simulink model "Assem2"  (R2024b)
settings: Solver=VariableStepAuto  StartTime=0.0  StopTime=10.0  RelTol=1e-3
undefined symbols (not defined in the file or in its folder): deg, kg, m, mm, N, s, smiData, X, Y, Z
libraries: sm_lib x14

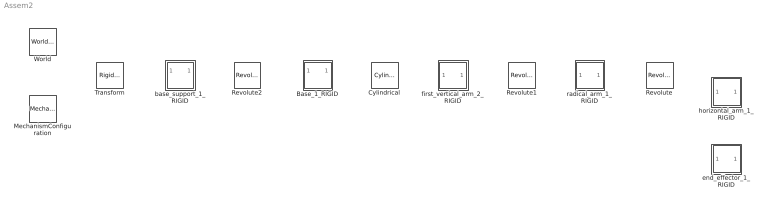
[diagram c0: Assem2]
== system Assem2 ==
  Base_1_RIGID : Subsystem
  Cylindrical : sm_lib/Joints/Cylindrical Joint  JointMode=Normal  CompositeWrenchDir=FollowerOnBase  CompositeWrenchFrame=BaseFrame  SenseConstraintForce=off  SenseConstraintTorque=off  SenseTotalForce=off  SenseTotalTorque=off  RzPositionTargetSpecify=on  RzPositionTargetPriority=Low  RzPositionTargetValue=smiData.CylindricalJoint(1).Rz.Pos  RzPositionTargetValueUnits=deg  RzVelocityTargetSpecify=off  RzVelocityTargetPriority=High  RzVelocityTargetValue=0  RzVelocityTargetValueUnits=deg/s  RzEquilibriumPosition=0  RzEquilibriumPositionUnits=deg  RzSpringStiffness=0  RzSpringStiffnessUnits=N*m/deg  RzDampingCoefficient=0  RzDampingCoefficientUnits=N*m/(deg/s)  RzLowerLimitSpecify=off  RzLowerLimitBound=-90  RzLowerLimitBoundUnits=deg  RzLowerLimitStiffness=1e4  RzLowerLimitStiffnessUnits=N*m/deg  RzLowerLimitDamping=10  RzLowerLimitDampingUnits=N*m/(deg/s)  RzLowerLimitTransitionRegionWidth=0.1  RzLowerLimitTransitionRegionWidthUnits=deg  RzUpperLimitSpecify=off  RzUpperLimitBound=90  RzUpperLimitBoundUnits=deg  RzUpperLimitStiffness=1e4  RzUpperLimitStiffnessUnits=N*m/deg  RzUpperLimitDamping=10  RzUpperLimitDampingUnits=N*m/(deg/s)  RzUpperLimitTransitionRegionWidth=0.1  RzUpperLimitTransitionRegionWidthUnits=deg  RzTorqueActuationMode=NoTorque  RzMotionActuationMode=ComputedMotion  RzSensePosition=off  RzSenseVelocity=off  RzSenseAcceleration=off  RzSenseTorqueForce=off  RzSenseLowerLimitTorqueForce=off  RzSenseUpperLimitTorqueForce=off  PzPositionTargetSpecify=on  PzPositionTargetPriority=Low  PzPositionTargetValue=smiData.CylindricalJoint(1).Pz.Pos  PzPositionTargetValueUnits=mm  PzVelocityTargetSpecify=off  PzVelocityTargetPriority=High  PzVelocityTargetValue=0  PzVelocityTargetValueUnits=m/s  PzEquilibriumPosition=0  PzEquilibriumPositionUnits=m  PzSpringStiffness=0  PzSpringStiffnessUnits=N/m  PzDampingCoefficient=0  PzDampingCoefficientUnits=N/(m/s)  PzLowerLimitSpecify=off  PzLowerLimitBound=-1  PzLowerLimitBoundUnits=m  PzLowerLimitStiffness=1e6  PzLowerLimitStiffnessUnits=N/m  PzLowerLimitDamping=1e3  PzLowerLimitDampingUnits=N/(m/s)  PzLowerLimitTransitionRegionWidth=1e-4  PzLowerLimitTransitionRegionWidthUnits=m  PzUpperLimitSpecify=off  PzUpperLimitBound=1  PzUpperLimitBoundUnits=m  PzUpperLimitStiffness=1e6  PzUpperLimitStiffnessUnits=N/m  PzUpperLimitDamping=1e3  PzUpperLimitDampingUnits=N/(m/s)  PzUpperLimitTransitionRegionWidth=1e-4  PzUpperLimitTransitionRegionWidthUnits=m  PzTorqueActuationMode=NoTorque  PzMotionActuationMode=ComputedMotion  PzSensePosition=off  PzSenseVelocity=off  PzSenseAcceleration=off  PzSenseTorqueForce=off  PzSenseLowerLimitTorqueForce=off  PzSenseUpperLimitTorqueForce=off
  MechanismConfiguration : sm_lib/Utilities/Mechanism Configuration  UniformGravity=Constant  GravityVector=[0 -9.80665 0]  GravityVectorUnits=m/s^2  LinearizationDelta=0.001  JointModeTransitionNonlinearIterations=2
  Revolute : sm_lib/Joints/Revolute Joint  JointMode=Normal  CompositeWrenchDir=FollowerOnBase  CompositeWrenchFrame=BaseFrame  SenseConstraintForce=off  SenseConstraintTorque=off  SenseTotalForce=off  SenseTotalTorque=off  PositionTargetSpecify=on  PositionTargetPriority=Low  PositionTargetValue=smiData.RevoluteJoint(1).Rz.Pos  PositionTargetValueUnits=deg  VelocityTargetSpecify=off  VelocityTargetPriority=High  VelocityTargetValue=0  VelocityTargetValueUnits=deg/s  EquilibriumPosition=0  EquilibriumPositionUnits=deg  SpringStiffness=0  SpringStiffnessUnits=N*m/deg  DampingCoefficient=0  DampingCoefficientUnits=N*m/(deg/s)  LowerLimitSpecify=off  LowerLimitBound=-90  LowerLimitBoundUnits=deg  LowerLimitStiffness=1e4  LowerLimitStiffnessUnits=N*m/deg  LowerLimitDamping=10  LowerLimitDampingUnits=N*m/(deg/s)  LowerLimitTransitionRegionWidth=0.1  LowerLimitTransitionRegionWidthUnits=deg  UpperLimitSpecify=off  UpperLimitBound=90  UpperLimitBoundUnits=deg  UpperLimitStiffness=1e4  UpperLimitStiffnessUnits=N*m/deg  UpperLimitDamping=10  UpperLimitDampingUnits=N*m/(deg/s)  UpperLimitTransitionRegionWidth=0.1  UpperLimitTransitionRegionWidthUnits=deg  TorqueActuationMode=NoTorque  MotionActuationMode=ComputedMotion  SensePosition=off  SenseVelocity=off  SenseAcceleration=off  SenseTorqueForce=off  SenseLowerLimitTorqueForce=off  SenseUpperLimitTorqueForce=off
  Revolute1 : sm_lib/Joints/Revolute Joint  JointMode=Normal  CompositeWrenchDir=FollowerOnBase  CompositeWrenchFrame=BaseFrame  SenseConstraintForce=off  SenseConstraintTorque=off  SenseTotalForce=off  SenseTotalTorque=off  PositionTargetSpecify=on  PositionTargetPriority=Low  PositionTargetValue=smiData.RevoluteJoint(2).Rz.Pos  PositionTargetValueUnits=deg  VelocityTargetSpecify=off  VelocityTargetPriority=High  VelocityTargetValue=0  VelocityTargetValueUnits=deg/s  EquilibriumPosition=0  EquilibriumPositionUnits=deg  SpringStiffness=0  SpringStiffnessUnits=N*m/deg  DampingCoefficient=0  DampingCoefficientUnits=N*m/(deg/s)  LowerLimitSpecify=off  LowerLimitBound=-90  LowerLimitBoundUnits=deg  LowerLimitStiffness=1e4  LowerLimitStiffnessUnits=N*m/deg  LowerLimitDamping=10  LowerLimitDampingUnits=N*m/(deg/s)  LowerLimitTransitionRegionWidth=0.1  LowerLimitTransitionRegionWidthUnits=deg  UpperLimitSpecify=off  UpperLimitBound=90  UpperLimitBoundUnits=deg  UpperLimitStiffness=1e4  UpperLimitStiffnessUnits=N*m/deg  UpperLimitDamping=10  UpperLimitDampingUnits=N*m/(deg/s)  UpperLimitTransitionRegionWidth=0.1  UpperLimitTransitionRegionWidthUnits=deg  TorqueActuationMode=NoTorque  MotionActuationMode=ComputedMotion  SensePosition=off  SenseVelocity=off  SenseAcceleration=off  SenseTorqueForce=off  SenseLowerLimitTorqueForce=off  SenseUpperLimitTorqueForce=off
  Revolute2 : sm_lib/Joints/Revolute Joint  JointMode=Normal  CompositeWrenchDir=FollowerOnBase  CompositeWrenchFrame=BaseFrame  SenseConstraintForce=off  SenseConstraintTorque=off  SenseTotalForce=off  SenseTotalTorque=off  PositionTargetSpecify=on  PositionTargetPriority=Low  PositionTargetValue=smiData.RevoluteJoint(3).Rz.Pos  PositionTargetValueUnits=deg  VelocityTargetSpecify=off  VelocityTargetPriority=High  VelocityTargetValue=0  VelocityTargetValueUnits=deg/s  EquilibriumPosition=0  EquilibriumPositionUnits=deg  SpringStiffness=0  SpringStiffnessUnits=N*m/deg  DampingCoefficient=0  DampingCoefficientUnits=N*m/(deg/s)  LowerLimitSpecify=off  LowerLimitBound=-90  LowerLimitBoundUnits=deg  LowerLimitStiffness=1e4  LowerLimitStiffnessUnits=N*m/deg  LowerLimitDamping=10  LowerLimitDampingUnits=N*m/(deg/s)  LowerLimitTransitionRegionWidth=0.1  LowerLimitTransitionRegionWidthUnits=deg  UpperLimitSpecify=off  UpperLimitBound=90  UpperLimitBoundUnits=deg  UpperLimitStiffness=1e4  UpperLimitStiffnessUnits=N*m/deg  UpperLimitDamping=10  UpperLimitDampingUnits=N*m/(deg/s)  UpperLimitTransitionRegionWidth=0.1  UpperLimitTransitionRegionWidthUnits=deg  TorqueActuationMode=NoTorque  MotionActuationMode=ComputedMotion  SensePosition=off  SenseVelocity=off  SenseAcceleration=off  SenseTorqueForce=off  SenseLowerLimitTorqueForce=off  SenseUpperLimitTorqueForce=off
  Transform : sm_lib/Frames and Transforms/Rigid Transform  RotationMethod=ArbitraryAxis  FollAlignAxisA=+X  BaseAlignAxisA=+Y  FollAlignAxisB=+Y  BaseAlignAxisB=+Z  RotationStandardAxis=+Z  RotationAngle=smiData.RigidTransform(21).angle  RotationAngleUnits=rad  RotationArbitraryAxis=smiData.RigidTransform(21).axis  RotationSequenceAxes=FollowerAxes  RotationSequence=XYX  RotationSequenceAngles=[0 0 0]  RotationSequenceAnglesUnits=deg  RotationMatrix=[1 0 0;0 1 0;0 0 1]  Quaternion=[1 0 0 0]  TranslationMethod=Cartesian  TranslationCartesianOffset=smiData.RigidTransform(21).translation  TranslationCartesianOffsetUnits=mm  TranslationStandardAxis=+Z  TranslationStandardOffset=0  TranslationStandardOffsetUnits=m  TranslationROffset=0  TranslationROffsetUnits=m  TranslationThetaOffset=0  TranslationThetaOffsetUnits=deg  TranslationZOffset=0  TranslationZOffsetUnits=m
  World : sm_lib/Frames and Transforms/World Frame
  base_support_1_RIGID : Subsystem
  end_effector_1_RIGID : Subsystem
  first_vertical_arm_2_RIGID : Subsystem
  horizontal_arm_1_RIGID : Subsystem
  radical_arm_1_RIGID : Subsystem

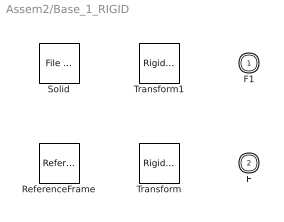
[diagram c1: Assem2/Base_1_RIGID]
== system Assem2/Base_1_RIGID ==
  ReferenceFrame : sm_lib/Frames and Transforms/Reference Frame
  Solid : sm_lib/Body Elements/File Solid  ExtGeomFileName=Base_Default_sldprt.STEP  UnitType=FromFile  ExtGeomFileUnits=m  StepReaderType=HEX  ExportConvexHullGeometry=off  InertiaType=Custom  BasedOnType=DensityFromFile  Density=1000  DensityUnits=kg/m^3  Mass=smiData.Solid(8).mass  MassUnits=kg  CenterOfMass=smiData.Solid(8).CoM  CenterOfMassUnits=mm  MomentsOfInertia=smiData.Solid(8).MoI  MomentsOfInertiaUnits=kg*mm^2  ProductsOfInertia=smiData.Solid(8).PoI  ProductsOfInertiaUnits=kg*mm^2  GraphicType=FromGeometry  MarkerShape=Sphere  MarkerSize=10  GraphicVisPropType=SimpleVisualProperties  GraphicDiffuseColor=smiData.Solid(8).color  GraphicOpacity=smiData.Solid(8).opacity  GraphicSpecularColor=[0.5 0.5 0.5 1.0]  GraphicAmbientColor=[0.15 0.15 0.15 1.0]  GraphicEmissiveColor=[0.0 0.0 0.0 1.0]  GraphicShininess=75  DoExposeReferenceFrame=on  SerializedFrames=<Frames/>
  Transform : sm_lib/Frames and Transforms/Rigid Transform  RotationMethod=ArbitraryAxis  FollAlignAxisA=+X  BaseAlignAxisA=+Y  FollAlignAxisB=+Y  BaseAlignAxisB=+Z  RotationStandardAxis=+Z  RotationAngle=smiData.RigidTransform(5).angle  RotationAngleUnits=rad  RotationArbitraryAxis=smiData.RigidTransform(5).axis  RotationSequenceAxes=FollowerAxes  RotationSequence=XYX  RotationSequenceAngles=[0 0 0]  RotationSequenceAnglesUnits=deg  RotationMatrix=[1 0 0;0 1 0;0 0 1]  Quaternion=[1 0 0 0]  TranslationMethod=Cartesian  TranslationCartesianOffset=smiData.RigidTransform(5).translation  TranslationCartesianOffsetUnits=mm  TranslationStandardAxis=+Z  TranslationStandardOffset=0  TranslationStandardOffsetUnits=m  TranslationROffset=0  TranslationROffsetUnits=m  TranslationThetaOffset=0  TranslationThetaOffsetUnits=deg  TranslationZOffset=0  TranslationZOffsetUnits=m
  Transform1 : sm_lib/Frames and Transforms/Rigid Transform  RotationMethod=ArbitraryAxis  FollAlignAxisA=+X  BaseAlignAxisA=+Y  FollAlignAxisB=+Y  BaseAlignAxisB=+Z  RotationStandardAxis=+Z  RotationAngle=smiData.RigidTransform(10).angle  RotationAngleUnits=rad  RotationArbitraryAxis=smiData.RigidTransform(10).axis  RotationSequenceAxes=FollowerAxes  RotationSequence=XYX  RotationSequenceAngles=[0 0 0]  RotationSequenceAnglesUnits=deg  RotationMatrix=[1 0 0;0 1 0;0 0 1]  Quaternion=[1 0 0 0]  TranslationMethod=Cartesian  TranslationCartesianOffset=smiData.RigidTransform(10).translation  TranslationCartesianOffsetUnits=mm  TranslationStandardAxis=+Z  TranslationStandardOffset=0  TranslationStandardOffsetUnits=m  TranslationROffset=0  TranslationROffsetUnits=m  TranslationThetaOffset=0  TranslationThetaOffsetUnits=deg  TranslationZOffset=0  TranslationZOffsetUnits=m
  F1 : PMIOPort  Side=Left
  F : PMIOPort  Port=2  Side=Right

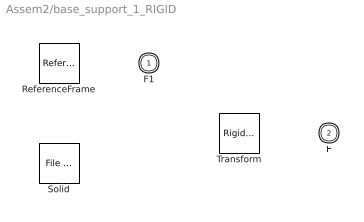
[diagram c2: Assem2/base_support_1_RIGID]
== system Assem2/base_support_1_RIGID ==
  ReferenceFrame : sm_lib/Frames and Transforms/Reference Frame
  Solid : sm_lib/Body Elements/File Solid  ExtGeomFileName=base support_Default_sldprt.STEP  UnitType=FromFile  ExtGeomFileUnits=m  StepReaderType=HEX  ExportConvexHullGeometry=off  InertiaType=Custom  BasedOnType=DensityFromFile  Density=1000  DensityUnits=kg/m^3  Mass=smiData.Solid(9).mass  MassUnits=kg  CenterOfMass=smiData.Solid(9).CoM  CenterOfMassUnits=mm  MomentsOfInertia=smiData.Solid(9).MoI  MomentsOfInertiaUnits=kg*mm^2  ProductsOfInertia=smiData.Solid(9).PoI  ProductsOfInertiaUnits=kg*mm^2  GraphicType=FromGeometry  MarkerShape=Sphere  MarkerSize=10  GraphicVisPropType=SimpleVisualProperties  GraphicDiffuseColor=smiData.Solid(9).color  GraphicOpacity=smiData.Solid(9).opacity  GraphicSpecularColor=[0.5 0.5 0.5 1.0]  GraphicAmbientColor=[0.15 0.15 0.15 1.0]  GraphicEmissiveColor=[0.0 0.0 0.0 1.0]  GraphicShininess=75  DoExposeReferenceFrame=on  SerializedFrames=<Frames/>
  Transform : sm_lib/Frames and Transforms/Rigid Transform  RotationMethod=ArbitraryAxis  FollAlignAxisA=+X  BaseAlignAxisA=+Y  FollAlignAxisB=+Y  BaseAlignAxisB=+Z  RotationStandardAxis=+Z  RotationAngle=smiData.RigidTransform(9).angle  RotationAngleUnits=rad  RotationArbitraryAxis=smiData.RigidTransform(9).axis  RotationSequenceAxes=FollowerAxes  RotationSequence=XYX  RotationSequenceAngles=[0 0 0]  RotationSequenceAnglesUnits=deg  RotationMatrix=[1 0 0;0 1 0;0 0 1]  Quaternion=[1 0 0 0]  TranslationMethod=Cartesian  TranslationCartesianOffset=smiData.RigidTransform(9).translation  TranslationCartesianOffsetUnits=mm  TranslationStandardAxis=+Z  TranslationStandardOffset=0  TranslationStandardOffsetUnits=m  TranslationROffset=0  TranslationROffsetUnits=m  TranslationThetaOffset=0  TranslationThetaOffsetUnits=deg  TranslationZOffset=0  TranslationZOffsetUnits=m
  F1 : PMIOPort  Side=Left
  F : PMIOPort  Port=2  Side=Right

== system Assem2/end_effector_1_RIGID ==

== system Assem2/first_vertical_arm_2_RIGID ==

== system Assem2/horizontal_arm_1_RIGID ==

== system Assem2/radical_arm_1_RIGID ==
